| IBIS file stm32wba62_a64_ufqfn48_usb.ibs
[IBIS ver] 4.2
[File name] stm32wba62_a64_ufqfn48_usb.ibs
[File Rev] 2.0
[Date] 17-02-2025
[Source] Data Created at STMicroelectronics
[Notes]  File originated from ELDO simulations.
[Disclaimer]  This information is for modeling purpose only and is
   not guaranted. The information is subject to change without
   notice.
[Copyright] Copyright 2025 STMicroelectronics Inc.
|   Component stm32wba62_a64_ufqfn48_usb
[Component] stm32wba62_a64_ufqfn48_usb
[Manufacturer] STMicroelectronics
[Package]
| variable   typ   min   max
R_pkg  0  NA  NA
L_pkg  0  NA  NA
C_pkg  0  NA  NA
[Pin]   signal_name   model_name
0  VSS  gnd
1  PB12  io8_ft_100m
2  PB11  io8_ft_100m_i2c
3  PA8  io8_ft_100m
4  PA7  io8_ft_100m_i2c_v33
5  PA6  io8_ft_100m_i2c
6  VDDA  nc
7  PA5  io8_ft_100m
8  PA3  io8_ft_100m
9  PB10  io8_ft_100m_i2c
10  PA2  io8_ft_100m_v33
11  VDD  power
12  PA1  io8_ft_100m
13  VDDUSB  power
14  PD9  io8_ft_100m
15  PD8  io8_ft_100m
16  PD7  io8_ft_100m
17  PD6  io8_ft_100m
18  PB8  io8_ft_100m
19  PC15-OSC32_OUT  io_ft_tamp
20  PC14-OSC32_IN  io_ft_tamp
21  PC13  io8_ft_100m_v33
22  VDD  power
23  PB4  io8_ft_100m
24  PB3  io8_ft_100m_i2c
25  PA15  io8_ft_100m_i2c
26  PA14  io8_ft_100m_v33
27  PA13  io8_ft_100m
28  PA12  io8_ft_100m
29  PA11  io8_ft_100m
30  PB2  io8_ft_100m_i2c_v33
31  PB1  io8_ft_100m_i2c
32  PB0  io8_ft_100m
33  PB15  io8_ft_100m
34  PH3-BOOT0  io8_ft_100m_v33
35  VDD  power
36  NRST  ioreset_v33
37  RF  nc
38  VDDHPA  nc
39  VDDRF  nc
40  OSC_OUT  nc
41  OSC_IN  nc
42  VDDRFPA  nc
43  VDD  power
44  VCAP  nc
45  PA10  io8_ft_100m
46  PA9  io8_ft_100m
47  PB14  io8_ft_100m_i2c
48  PB13  io8_ft_100m_i2c
[Package Model]   4b0-ufqfn-7x7-48-250115
[Pin Mapping]   pulldown_ref   pullup_ref   | Comment
0  gndio  nc
1  gndio  vddio
2  gndio  vddio
3  gndio  vddio
4  gndio  vddio
5  gndio  vddio
6  nc  nc
7  gndio  vddio
8  gndio  vddio
9  gndio  vddio
10  gndio  vddio
11  nc  vddio
12  gndio  vddio
13  nc  vddusb
14  gndio  vddio  | Depending on IO usage
| 14  gndio  vddusb  | Depending on IO usage
15  gndio  vddio  | Depending on IO usage
| 15  gndio  vddusb  | Depending on IO usage
16  gndio  vddio
17  gndio  vddio
18  gndio  vddio
19  gndio  vddio
20  gndio  vddio
21  gndio  vddio
22  nc  vddio
23  gndio  vddio
24  gndio  vddio
25  gndio  vddio
26  gndio  vddio
27  gndio  vddio
28  gndio  vddio
29  gndio  vddio
30  gndio  vddio
31  gndio  vddio
32  gndio  vddio
33  gndio  vddio
34  gndio  vddio
35  nc  vddio
36  gndio  vddio
37  nc  nc
38  nc  nc
39  nc  nc
40  nc  nc
41  nc  nc
42  nc  nc
43  nc  vddio
44  nc  nc
45  gndio  vddio
46  gndio  vddio
47  gndio  vddio
48  gndio  vddio
|[Diff Pin]  inv_pin  vdiff  tdelay_typ  tdelay_min  tdelay_max
|17  16  NA  NA  NA  NA
[Model Selector] io8_ft_100m
io8_ft_100m_ls_1v2  "GPIO 100MHz - 5V tolerant - low speed - 1.2V range"
io8_ft_100m_ls_1v8  "GPIO 100MHz - 5V tolerant - low speed - 1.8V range"
io8_ft_100m_ls_3v3  "GPIO 100MHz - 5V tolerant - low speed - 3.3V range"
io8_ft_100m_ms_1v2  "GPIO 100MHz - 5V tolerant - med speed - 1.2V range"
io8_ft_100m_ms_1v8  "GPIO 100MHz - 5V tolerant - med speed - 1.8V range"
io8_ft_100m_ms_3v3  "GPIO 100MHz - 5V tolerant - med speed - 3.3V range"
io8_ft_100m_fs_1v2  "GPIO 100MHz - 5V tolerant - fast speed - 1.2V range"
io8_ft_100m_fs_1v8  "GPIO 100MHz - 5V tolerant - fast speed - 1.8V range"
io8_ft_100m_fs_3v3  "GPIO 100MHz - 5V tolerant - fast speed - 3.3V range"
io8_ft_100m_hs_1v2  "GPIO 100MHz - 5V tolerant - high speed - 1.2V range"
io8_ft_100m_hs_1v8  "GPIO 100MHz - 5V tolerant - high speed - 1.8V range"
io8_ft_100m_hs_3v3  "GPIO 100MHz - 5V tolerant - high speed - 3.3V range"
[Model Selector] io8_ft_100m_i2c
io8_ft_100m_ls_1v2  "GPIO 100MHz - 5V tolerant - low speed - 1.2V range"
io8_ft_100m_ls_1v8  "GPIO 100MHz - 5V tolerant - low speed - 1.8V range"
io8_ft_100m_ls_3v3  "GPIO 100MHz - 5V tolerant - low speed - 3.3V range"
io8_ft_100m_ms_1v2  "GPIO 100MHz - 5V tolerant - med speed - 1.2V range"
io8_ft_100m_ms_1v8  "GPIO 100MHz - 5V tolerant - med speed - 1.8V range"
io8_ft_100m_ms_3v3  "GPIO 100MHz - 5V tolerant - med speed - 3.3V range"
io8_ft_100m_fs_1v2  "GPIO 100MHz - 5V tolerant - fast speed - 1.2V range"
io8_ft_100m_fs_1v8  "GPIO 100MHz - 5V tolerant - fast speed - 1.8V range"
io8_ft_100m_fs_3v3  "GPIO 100MHz - 5V tolerant - fast speed - 3.3V range"
io8_ft_100m_hs_1v2  "GPIO 100MHz - 5V tolerant - high speed - 1.2V range"
io8_ft_100m_hs_1v8  "GPIO 100MHz - 5V tolerant - high speed - 1.8V range"
io8_ft_100m_hs_3v3  "GPIO 100MHz - 5V tolerant - high speed - 3.3V range"
io8_ft_100m_i2c_ls_1v2  "GPIO 100MHz with I2C open-drain - 5V tolerant - low speed - 1.2V range"
io8_ft_100m_i2c_ls_1v8  "GPIO 100MHz with I2C open-drain - 5V tolerant - low speed - 1.8V range"
io8_ft_100m_i2c_ls_3v3  "GPIO 100MHz with I2C open-drain - 5V tolerant - low speed - 3.3V range"
io8_ft_100m_i2c_ms_1v2  "GPIO 100MHz with I2C open-drain - 5V tolerant - med speed - 1.2V range"
io8_ft_100m_i2c_ms_1v8  "GPIO 100MHz with I2C open-drain - 5V tolerant - med speed - 1.8V range"
io8_ft_100m_i2c_ms_3v3  "GPIO 100MHz with I2C open-drain - 5V tolerant - med speed - 3.3V range"
io8_ft_100m_i2c_fs_1v2  "GPIO 100MHz with I2C open-drain - 5V tolerant - fast speed - 1.2V range"
io8_ft_100m_i2c_fs_1v8  "GPIO 100MHz with I2C open-drain - 5V tolerant - fast speed - 1.8V range"
io8_ft_100m_i2c_fs_3v3  "GPIO 100MHz with I2C open-drain - 5V tolerant - fast speed - 3.3V range"
io8_ft_100m_i2c_hs_1v2  "GPIO 100MHz with I2C open-drain - 5V tolerant - high speed - 1.2V range"
io8_ft_100m_i2c_hs_1v8  "GPIO 100MHz with I2C open-drain - 5V tolerant - high speed - 1.8V range"
io8_ft_100m_i2c_hs_3v3  "GPIO 100MHz with I2C open-drain - 5V tolerant - high speed - 3.3V range"
io8_ft_100m_i2c_fmp_3v3  "GPIO 100MHz with I2C fm+ open-drain - 5V tolerant - low speed - 3.3V range"
io8_ft_100m_i2c_fmp_1v8  "GPIO 100MHz with I2C fm+ open-drain - 5V tolerant - low speed - 1.8V range"
io8_ft_100m_i2c_fmp_1v2  "GPIO 100MHz with I2C fm+ open-drain - 5V tolerant - low speed - 1.2V range"
[Model Selector] io8_ft_100m_i2c_v33
io8_ft_100m_v33_ls_1v2  "GPIO_V33 100MHz - 5V tolerant - low speed - 1.2V range"
io8_ft_100m_v33_ls_1v8  "GPIO_V33 100MHz - 5V tolerant - low speed - 1.8V range"
io8_ft_100m_v33_ls_3v3  "GPIO_V33 100MHz - 5V tolerant - low speed - 3.3V range"
io8_ft_100m_v33_ms_1v2  "GPIO_V33 100MHz - 5V tolerant - med speed - 1.2V range"
io8_ft_100m_v33_ms_1v8  "GPIO_V33 100MHz - 5V tolerant - med speed - 1.8V range"
io8_ft_100m_v33_ms_3v3  "GPIO_V33 100MHz - 5V tolerant - med speed - 3.3V range"
io8_ft_100m_v33_fs_1v2  "GPIO_V33 100MHz - 5V tolerant - fast speed - 1.2V range"
io8_ft_100m_v33_fs_1v8  "GPIO_V33 100MHz - 5V tolerant - fast speed - 1.8V range"
io8_ft_100m_v33_fs_3v3  "GPIO_V33 100MHz - 5V tolerant - fast speed - 3.3V range"
io8_ft_100m_v33_hs_1v2  "GPIO_V33 100MHz - 5V tolerant - high speed - 1.2V range"
io8_ft_100m_v33_hs_1v8  "GPIO_V33 100MHz - 5V tolerant - high speed - 1.8V range"
io8_ft_100m_v33_hs_3v3  "GPIO_V33 100MHz - 5V tolerant - high speed - 3.3V range"
io8_ft_100m_i2c_v33_ls_1v2  "GPIO_V33 100MHz with I2C open-drain - 5V tolerant - low speed - 1.2V range"
io8_ft_100m_i2c_v33_ls_1v8  "GPIO_V33 100MHz with I2C open-drain - 5V tolerant - low speed - 1.8V range"
io8_ft_100m_i2c_v33_ls_3v3  "GPIO_V33 100MHz with I2C open-drain - 5V tolerant - low speed - 3.3V range"
io8_ft_100m_i2c_v33_ms_1v2  "GPIO_V33 100MHz with I2C open-drain - 5V tolerant - med speed - 1.2V range"
io8_ft_100m_i2c_v33_ms_1v8  "GPIO_V33 100MHz with I2C open-drain - 5V tolerant - med speed - 1.8V range"
io8_ft_100m_i2c_v33_ms_3v3  "GPIO_V33 100MHz with I2C open-drain - 5V tolerant - med speed - 3.3V range"
io8_ft_100m_i2c_v33_fs_1v2  "GPIO_V33 100MHz with I2C open-drain - 5V tolerant - fast speed - 1.2V range"
io8_ft_100m_i2c_v33_fs_1v8  "GPIO_V33 100MHz with I2C open-drain - 5V tolerant - fast speed - 1.8V range"
io8_ft_100m_i2c_v33_fs_3v3  "GPIO_V33 100MHz with I2C open-drain - 5V tolerant - fast speed - 3.3V range"
io8_ft_100m_i2c_v33_hs_1v2  "GPIO_V33 100MHz with I2C open-drain - 5V tolerant - high speed - 1.2V range"
io8_ft_100m_i2c_v33_hs_1v8  "GPIO_V33 100MHz with I2C open-drain - 5V tolerant - high speed - 1.8V range"
io8_ft_100m_i2c_v33_hs_3v3  "GPIO_V33 100MHz with I2C open-drain - 5V tolerant - high speed - 3.3V range"
io8_ft_100m_i2c_fmp_v33_1v2  "GPIO_V33 100MHz with I2C fm+ open-drain - 5V tolerant - low speed - 1.2V range"
io8_ft_100m_i2c_fmp_v33_1v8  "GPIO_V33 100MHz with I2C fm+ open-drain - 5V tolerant - low speed - 1.8V range"
io8_ft_100m_i2c_fmp_v33_3v3  "GPIO_V33 100MHz with I2C fm+ open-drain - 5V tolerant - low speed - 3.3V range"
[Model Selector] io8_ft_100m_v33
io8_ft_100m_v33_ls_1v2  "GPIO_V33 100MHz - 5V tolerant - low speed - 1.2V range"
io8_ft_100m_v33_ls_1v8  "GPIO_V33 100MHz - 5V tolerant - low speed - 1.8V range"
io8_ft_100m_v33_ls_3v3  "GPIO_V33 100MHz - 5V tolerant - low speed - 3.3V range"
io8_ft_100m_v33_ms_1v2  "GPIO_V33 100MHz - 5V tolerant - med speed - 1.2V range"
io8_ft_100m_v33_ms_1v8  "GPIO_V33 100MHz - 5V tolerant - med speed - 1.8V range"
io8_ft_100m_v33_ms_3v3  "GPIO_V33 100MHz - 5V tolerant - med speed - 3.3V range"
io8_ft_100m_v33_fs_1v2  "GPIO_V33 100MHz - 5V tolerant - fast speed - 1.2V range"
io8_ft_100m_v33_fs_1v8  "GPIO_V33 100MHz - 5V tolerant - fast speed - 1.8V range"
io8_ft_100m_v33_fs_3v3  "GPIO_V33 100MHz - 5V tolerant - fast speed - 3.3V range"
io8_ft_100m_v33_hs_1v2  "GPIO_V33 100MHz - 5V tolerant - high speed - 1.2V range"
io8_ft_100m_v33_hs_1v8  "GPIO_V33 100MHz - 5V tolerant - high speed - 1.8V range"
io8_ft_100m_v33_hs_3v3  "GPIO_V33 100MHz - 5V tolerant - high speed - 3.3V range"
[Model Selector] io_ft_tamp
io_ft_tamp_ls_1v2 "io8_ft tamp low speed @ 1.2V"
io_ft_tamp_ls_1v8 "io8_ft tamp low speed @ 1.8V"
io_ft_tamp_ls_3v3 "io8_ft tamp low speed @ 3.3V"
io_ft_tamp_ms_1v2 "io8_ft tamp med speed @ 1.2V"
io_ft_tamp_ms_1v8 "io8_ft tamp med speed @ 1.8V"
io_ft_tamp_ms_3v3 "io8_ft tamp med speed @ 3.3V"
io_ft_tamp_fs_1v2 "io8_ft tamp fast speed @ 1.2V"
io_ft_tamp_fs_1v8 "io8_ft tamp fast speed @ 1.8V"
io_ft_tamp_fs_3v3 "io8_ft tamp fast speed @ 3.3V"
io_ft_tamp_hs_1v2 "io8_ft tamp high speed @ 1.2V"
io_ft_tamp_hs_1v8 "io8_ft tamp high speed @ 1.8V"
io_ft_tamp_hs_3v3 "io8_ft tamp high speed @ 3.3V"
[Model Selector] ioreset_v33
ioreset_v33_1v2 "Reset PAD. 5V tolerant. 1.2V range"
ioreset_v33_1v8 "Reset PAD. 5V tolerant. 1.8V range"
ioreset_v33_3v3 "Reset PAD. 5V tolerant. 3.3V range"
[Define Package Model]  4b0-ufqfn-7x7-48-250115
[Manufacturer]  Unknown
[OEM]  Unknown
[Description]  None
[Number Of Pins]  49
[Pin Numbers]
| Pin Num   Terminal Name
36 | NRST
41 | OSC_IN
40 | OSC_OUT
12 | PA1
10 | PA2
8 | PA3
7 | PA5
5 | PA6
4 | PA7
3 | PA8
46 | PA9
45 | PA10
29 | PA11
28 | PA12
27 | PA13
26 | PA14
25 | PA15
32 | PB0
31 | PB1
30 | PB2
24 | PB3
23 | PB4
18 | PB8
9 | PB10
2 | PB11
1 | PB12
48 | PB13
47 | PB14
33 | PB15
21 | PC13
20 | PC14-OSC32_IN
19 | PC15-OSC32_OUT
17 | PD6
16 | PD7
15 | PD8
14 | PD9
34 | PH3-BOOT0
37 | RF
44 | VCAP
22 | VDD
35 | VDD
43 | VDD
6 | VDDA
38 | VDDHPA
11 | VDD
39 | VDDRF
42 | VDDRFPA
13 | VDDUSB
0 | VSS
[Model Data]
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[End Model Data]
[End Package Model]
|End [Component]
| Models and submodels in the file (69): io8_ft_100m_fs_1v2 (I/O), io8_ft_100m_fs_1v8 (I/O), io8_ft_100m_fs_3v3 (I/O), io8_ft_100m_hs_1v2 (I/O), io8_ft_100m_hs_1v8 (I/O), io8_ft_100m_hs_3v3 (I/O), io8_ft_100m_i2c_fmp_1v2 (I/O_open_drain), io8_ft_100m_i2c_fmp_1v8 (I/O_open_drain), io8_ft_100m_i2c_fmp_3v3 (I/O_open_drain), io8_ft_100m_i2c_fmp_v33_1v2 (I/O_open_drain), io8_ft_100m_i2c_fmp_v33_1v8 (I/O_open_drain), io8_ft_100m_i2c_fmp_v33_3v3 (I/O_open_drain), io8_ft_100m_i2c_fs_1v2 (I/O_open_drain), io8_ft_100m_i2c_fs_1v8 (I/O_open_drain), io8_ft_100m_i2c_fs_3v3 (I/O_open_drain), io8_ft_100m_i2c_hs_1v2 (I/O_open_drain), io8_ft_100m_i2c_hs_1v8 (I/O_open_drain), io8_ft_100m_i2c_hs_3v3 (I/O_open_drain), io8_ft_100m_i2c_ls_1v2 (I/O_open_drain), io8_ft_100m_i2c_ls_1v8 (I/O_open_drain), io8_ft_100m_i2c_ls_3v3 (I/O_open_drain), io8_ft_100m_i2c_ms_1v2 (I/O_open_drain), io8_ft_100m_i2c_ms_1v8 (I/O_open_drain), io8_ft_100m_i2c_ms_3v3 (I/O_open_drain), io8_ft_100m_i2c_v33_fs_1v2 (I/O_open_drain), io8_ft_100m_i2c_v33_fs_1v8 (I/O_open_drain), io8_ft_100m_i2c_v33_fs_3v3 (I/O_open_drain), io8_ft_100m_i2c_v33_hs_1v2 (I/O_open_drain), io8_ft_100m_i2c_v33_hs_1v8 (I/O_open_drain), io8_ft_100m_i2c_v33_hs_3v3 (I/O_open_drain), io8_ft_100m_i2c_v33_ls_1v2 (I/O_open_drain), io8_ft_100m_i2c_v33_ls_1v8 (I/O_open_drain), io8_ft_100m_i2c_v33_ls_3v3 (I/O_open_drain), io8_ft_100m_i2c_v33_ms_1v2 (I/O_open_drain), io8_ft_100m_i2c_v33_ms_1v8 (I/O_open_drain), io8_ft_100m_i2c_v33_ms_3v3 (I/O_open_drain), io8_ft_100m_ls_1v2 (I/O), io8_ft_100m_ls_1v8 (I/O), io8_ft_100m_ls_3v3 (I/O), io8_ft_100m_ms_1v2 (I/O), io8_ft_100m_ms_1v8 (I/O), io8_ft_100m_ms_3v3 (I/O), io8_ft_100m_v33_fs_1v2 (I/O), io8_ft_100m_v33_fs_1v8 (I/O), io8_ft_100m_v33_fs_3v3 (I/O), io8_ft_100m_v33_hs_1v2 (I/O), io8_ft_100m_v33_hs_1v8 (I/O), io8_ft_100m_v33_hs_3v3 (I/O), io8_ft_100m_v33_ls_1v2 (I/O), io8_ft_100m_v33_ls_1v8 (I/O), io8_ft_100m_v33_ls_3v3 (I/O), io8_ft_100m_v33_ms_1v2 (I/O), io8_ft_100m_v33_ms_1v8 (I/O), io8_ft_100m_v33_ms_3v3 (I/O), io_ft_tamp_fs_1v2 (I/O), io_ft_tamp_fs_1v8 (I/O), io_ft_tamp_fs_3v3 (I/O), io_ft_tamp_hs_1v2 (I/O), io_ft_tamp_hs_1v8 (I/O), io_ft_tamp_hs_3v3 (I/O), io_ft_tamp_ls_1v2 (I/O), io_ft_tamp_ls_1v8 (I/O), io_ft_tamp_ls_3v3 (I/O), io_ft_tamp_ms_1v2 (I/O), io_ft_tamp_ms_1v8 (I/O), io_ft_tamp_ms_3v3 (I/O), ioreset_v33_1v2 (I/O_open_drain), ioreset_v33_1v8 (I/O_open_drain), ioreset_v33_3v3 (I/O_open_drain)
